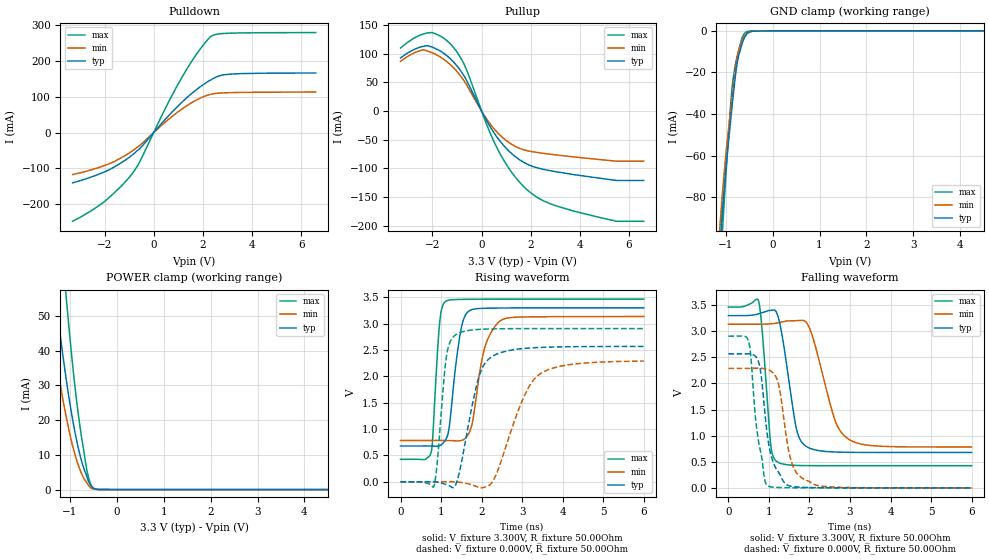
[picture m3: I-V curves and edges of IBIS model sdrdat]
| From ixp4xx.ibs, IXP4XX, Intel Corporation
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[Model]   sdrdat
Model_type   I/O
Vinl = 800.000mV
Vinh = 2.000V
Vmeas = 1.500V
Cref = 0.000F
|   typ   min   max
C_comp   3.000pF   2.700pF   3.300pF
[Voltage Range]   3.300V   3.135V   3.465V
[Temperature Range]   25.0   110.0   -40.0
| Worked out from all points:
|   slope of the pulldown table from 0 to 0.495 V, typ, clamps not added: 12.8 ohm
|   slope of the pullup table from 0 to 0.495 V, typ, clamps not added: 13.3 ohm
|   GND clamp passes 1 mA (typ) near -0.52 V on its own axis
|   POWER clamp passes 1 mA (typ) near -0.54 V on its own axis
|   falling waveform, V_fixture 3.300V, R_fixture 50.00Ohm: 20-80 % time 303ps typ, 487ps min, 170ps max; typ from 3.3 V to 0.679 V
|   rising waveform, V_fixture 3.300V, R_fixture 50.00Ohm: 20-80 % time 239ps typ, 327ps min, 138ps max; typ from 0.679 V to 3.3 V
|   rising waveform, V_fixture 0.000V, R_fixture 50.00Ohm: 20-80 % time 421ps typ, 681ps min, 194ps max; typ from 0 V to 2.57 V
|   falling waveform, V_fixture 0.000V, R_fixture 50.00Ohm: 20-80 % time 273ps typ, 297ps min, 248ps max; typ from 2.57 V to 0 V
[Pulldown]
|   Voltage   I(typ)   I(min)   I(max)
-3.3V     -140.8mA   -117.5mA   -248.5mA
-2.045V   -111.4mA   -93.32mA   -195.4mA
-1.35V    -85.8mA    -71.71mA   -151.9mA
-865mV    -62.42mA   -51.19mA   -114mA
-595mV    -46.76mA   -37.67mA   -85.4mA
380mV     30.08mA    23.84mA    54.56mA
1.11V     82.34mA    64.03mA    149.9mA
1.73V     119.6mA    90.68mA    218.3mA
2.3V      146.6mA    106.9mA    267.6mA
2.645V    158.4mA    110.3mA    276.1mA
3.12V     163.6mA    111.8mA    278.3mA
6.595V    166.9mA    113.5mA    280mA
[GND Clamp]
|   Voltage   I(typ)   I(min)   I(max)
-3.3V     -1.926A    -1.857A    -2.229A
-1.125V   -104.7mA   -94.64mA   -120.7mA
-1.07V    -87.27mA   -78.33mA   -96.87mA
-1.055V   -82.72mA   -74.31mA   -91.06mA
-945mV    -54.52mA   -48.52mA   -52.01mA
-885mV    -41.01mA   -36.18mA   -32.8mA
-845mV    -32.21mA   -28.33mA   -23.45mA
-780mV    -19.26mA   -16.38mA   -14.82mA
-730mV    -12.61mA   -9.931mA   -10.3mA
-645mV    -5.855mA   -4.483mA   -3.098mA
-555mV    -1.736mA   -1.231mA   -418.7uA
6.595V    0A         0A         0A
[Pullup]
|   Voltage   I(typ)   I(min)   I(max)
-3.3V     92.63mA    86.76mA    110mA
-2.47V    111.8mA    105.7mA    132.9mA
-2.035V   111.7mA    102mA      136.8mA
-1.19V    87.67mA    77.47mA    113.2mA
-680mV    58.66mA    50.54mA    78.65mA
240mV     -19.41mA   -16mA      -27.15mA
795mV     -54.7mA    -43.85mA   -77.66mA
1.42V     -81.01mA   -62.49mA   -117.7mA
2.125V    -97.16mA   -71.21mA   -146.4mA
3.03V     -105.8mA   -76.44mA   -165.1mA
4.675V    -116.2mA   -83.9mA    -184mA
6.595V    -121mA     -87.39mA   -192mA
[POWER Clamp]
|   Voltage   I(typ)   I(min)   I(max)
-3.3V     403.8mA    324.6mA    607.2mA
-1.515V   82.48mA    59.25mA    137.1mA
-1.465V   75.77mA    54.07mA    126.5mA
-1.31V    56.36mA    39.24mA    95.65mA
-1.09V    32.91mA    21.77mA    57.38mA
-1.06V    30.12mA    19.75mA    52.74mA
-935mV    19.72mA    12.33mA    35.15mA
-785mV    10.02mA    5.771mA    18.26mA
-635mV    3.649mA    1.937mA    5.465mA
-530mV    782.2uA    338.8uA    898uA
-390mV    54.09uA    21.66uA    23.63uA
6.595V    0A         0A         0A
[Ramp]
R_load = 50.00Ohm
|   typ   min   max
dV/dt_r   1.540V/420.589ps   1.374V/680.349ps   1.744V/193.462ps
dV/dt_f   1.573V/302.862ps   1.411V/486.967ps   1.824V/170.153ps
[Falling Waveform]
V_fixture = 3.300V
V_fixture_min = 3.135V
V_fixture_max = 3.465V
R_fixture = 50.00Ohm
|   Time   V(typ)   V(min)   V(max)
0s        3.3V       3.135V     3.465V
740ps     3.334V     3.135V     3.588V
830ps     3.357V     3.136V     3.035V
1.05ns    3.402V     3.144V     784.5mV
1.21ns    3.316V     3.16V      496mV
1.68ns    1.123V     3.204V     430.3mV
1.91ns    800.1mV    3.18V      426.6mV
2.62ns    687.4mV    1.317V     424.9mV
2.91ns    681.9mV    962.5mV    424.9mV
6ns       678.8mV    782.9mV    424.9mV
[Rising Waveform]
V_fixture = 3.300V
V_fixture_min = 3.135V
V_fixture_max = 3.465V
R_fixture = 50.00Ohm
|   Time   V(typ)   V(min)   V(max)
0s        678.8mV    782.9mV    424.9mV
750ps     677.6mV    783.3mV    543.5mV
960ps     682.7mV    783.7mV    2.976V
1.12ns    806.1mV    782.5mV    3.426V
1.2ns     1.029V     781.1mV    3.447V
1.49ns    2.88V      781mV      3.46V
1.71ns    3.249V     958.9mV    3.462V
2.06ns    3.291V     2.493V     3.464V
2.45ns    3.296V     3.047V     3.465V
6ns       3.3V       3.135V     3.465V
[Rising Waveform]
V_fixture = 0.000V
V_fixture_min = 0.000V
V_fixture_max = 0.000V
R_fixture = 50.00Ohm
|   Time   V(typ)   V(min)   V(max)
0s        983.4nV    357.6nV    25.21nV
820ps     -1.614mV   -41.26uV   -96.09mV
900ps     -9.926mV   102.3uV    318.3mV
1.13ns    -53.64mV   874.6uV    2.362V
1.38ns    -18.51mV   -3.405mV   2.797V
1.9ns     1.896V     -99.36mV   2.889V
2.22ns    2.355V     -48.22mV   2.9V
3ns       2.525V     1.532V     2.905V
3.4ns     2.547V     2.021V     2.906V
6ns       2.567V     2.29V      2.906V
[Falling Waveform]
V_fixture = 0.000V
V_fixture_min = 0.000V
V_fixture_max = 0.000V
R_fixture = 50.00Ohm
|   Time   V(typ)   V(min)   V(max)
0s        2.567V     2.29V      2.906V
500ps     2.57V      2.29V      2.798V
670ps     2.517V     2.292V     1.324V
770ps     2.335V     2.293V     781.3mV
970ps     954.3mV    2.267V     37.74mV
1.21ns    326mV      2.056V     8.176mV
1.36ns    120.2mV    1.366V     4.24mV
1.57ns    27.33mV    461.3mV    1.589mV
1.85ns    10.11mV    172.2mV    395uV
6ns       983.4nV    357.6nV    25.21nV
